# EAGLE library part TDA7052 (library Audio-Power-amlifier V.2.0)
1 W BTL mono audio amplifier Source : www.datasheetcatalog.org/datasheet/philips/TDA7052_CNV_2.pdf
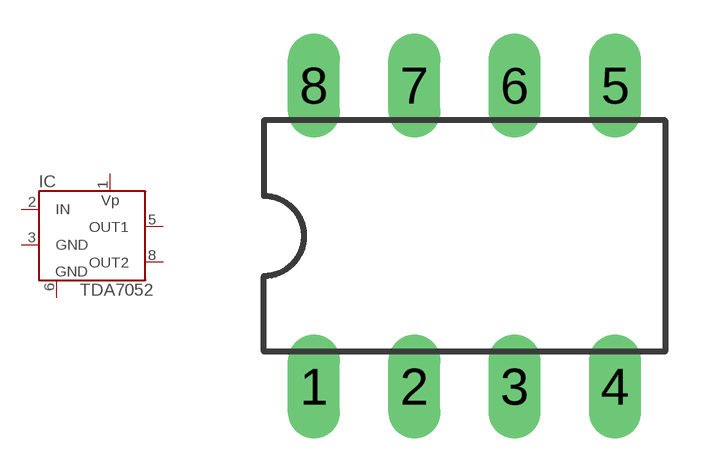
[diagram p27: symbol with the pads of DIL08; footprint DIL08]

Designator prefix IC

## TDA7052  [DIL08]
1  VP  sup
2  IN  in
3  GND  sup
5  OUT1  out
6  GND  sup
8  OUT2  out

## Footprint DIL08 (pad centres in mm)
Dual In Line Package
drill 0.813 pad 1.27 long: 1 -3.81,-3.81; 2 -1.27,-3.81; 3 1.27,-3.81; 4 3.81,-3.81; 5 3.81,3.81; 6 1.27,3.81; 7 -1.27,3.81; 8 -3.81,3.81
